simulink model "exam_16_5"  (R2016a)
settings: Solver=ode45  StartTime=0.0  StopTime=0.1  MaxStep=0.0005  RelTol=1e-3

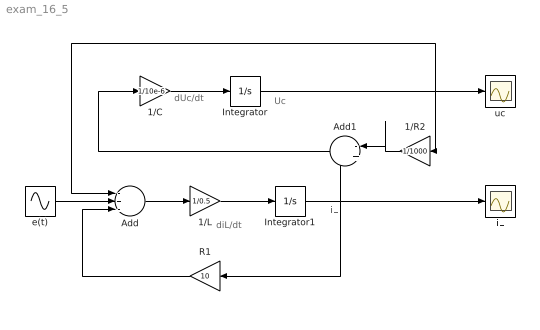
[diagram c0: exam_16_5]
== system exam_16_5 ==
  note: iL
  note: Uc
  note: diL/dt
  note: dUc/dt
  1/C : Gain  Gain=1/10e-6
  1/L : Gain  Gain=1/0.5
  1/R2 : Gain  Gain=1/1000
  Add : Sum  Inputs=-+-
  Add1 : Sum  Inputs=-+  RndMeth=Zero
  Integrator : Integrator
  Integrator1 : Integrator
  R1 : Gain  Gain=10
  e(t) : Sin  Amplitude=100*sqrt(2)  Frequency=2*pi*50  SampleTime=0
  iL : Scope
  uc : Scope
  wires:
  1/L/1 -> Integrator1/1
  Integrator/1 -> 1/R2/1, uc/1, Add/1
  Integrator1/1 -> Add1/2, iL/1, R1/1
  Add/1 -> 1/L/1
  e(t)/1 -> Add/2
  R1/1 -> Add/3
  1/R2/1 -> Add1/1
  1/C/1 -> Integrator/1
  Add1/1 -> 1/C/1
